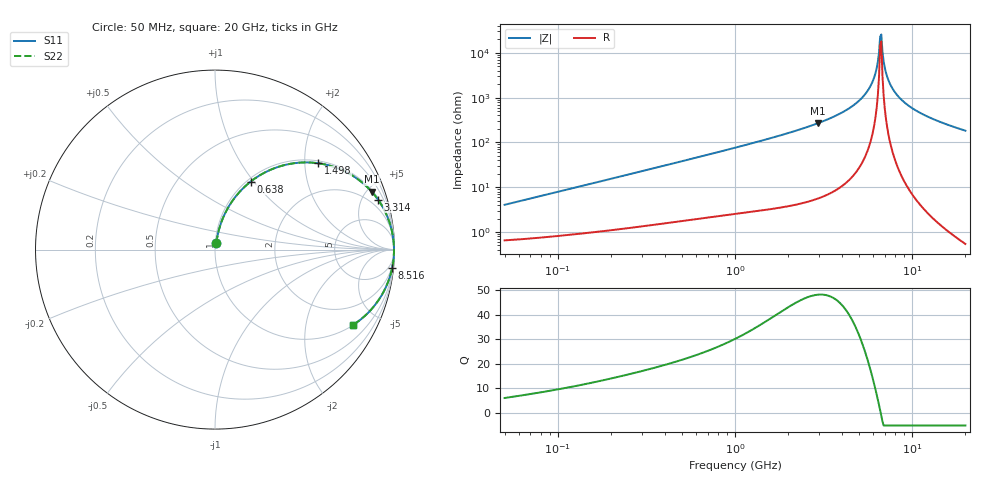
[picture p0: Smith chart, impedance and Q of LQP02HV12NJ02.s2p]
!Murata Part Number: LQP02HV12NJ02
!These Parameters are Measured in Series Mode Connection
!  o--[Z]--o
!Port1  Port2
!  o-------o
!Freq. Start=50[MHz] Stop=20[GHz], 401[Steps]
# Hz S RI R 50
!Freq.(Hz) S11(Real) S11(Imag) S21(Real) S21(Imag) S12(Real) S12(Imag) S22(Real) S22(Imag)
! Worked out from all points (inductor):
!   401 points, 50 MHz to 20 GHz, reference 50 ohm
!   read as one part in series: L = 12.6 nH near 51.52 MHz
!   highest Q = 48.1 at 2.94 GHz (marker M1), where L = 14.5 nH
!   self-resonance near 6.602 GHz
!   S11 on the Smith chart (normalised r, x): 50 MHz: 1.01, +0.08; 638 MHz: 1.04, +0.96; 1.498 GHz: 1.06, +2.33; 3.314 GHz: 1.14, +6.47; 8.516 GHz: 1, -20; 20 GHz: 1.01, -3.65
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5e7  0.00803 0.0394  0.992 -0.0394  0.992 -0.0394  0.00803 0.0394
1.364002e8  0.02 0.1031  0.98 -0.1031  0.98 -0.1031  0.02 0.1031
3.721004e8  0.0858 0.2549  0.9142 -0.2549  0.9142 -0.2549  0.0858 0.2549
6.380365e8  0.1987 0.3789  0.8013 -0.3789  0.8013 -0.3789  0.1987 0.3789
1e9  0.3704 0.4666  0.6296 -0.4666  0.6296 -0.4666  0.3704 0.4666
1.498439e9  0.5742 0.4812  0.4258 -0.4812  0.4258 -0.4812  0.5742 0.4812
2.728004e9  0.8479 0.3487  0.1521 -0.3487  0.1521 -0.3487  0.8479 0.3487
2.940159e9  0.873 0.3227  0.127 -0.3227  0.127 -0.3227  0.873 0.3227
3.314454e9  0.908 0.2787  0.092 -0.2787  0.092 -0.2787  0.908 0.2787
4.539627e9  0.971 0.1552  0.029 -0.1552  0.029 -0.1552  0.971 0.1552
5.515528e9  0.9908 0.0765  0.00922 -0.0765  0.00922 -0.0765  0.9908 0.0765
5.856089e9  0.9942 0.0521  0.00584 -0.0521  0.00584 -0.0521  0.9942 0.0521
6.125241e9  0.9959 0.0338  0.00412 -0.0338  0.00412 -0.0338  0.9959 0.0338
6.311513e9  0.9966 0.0217  0.00336 -0.0217  0.00336 -0.0217  0.9966 0.0217
6.503449e9  0.9971 0.00945  0.0029 -0.00945  0.0029 -0.00945  0.9971 0.00945
6.601595e9  0.9972 0.00335  0.00278 -0.00335  0.00278 -0.00335  0.9972 0.00335
6.802353e9  0.9972 -0.00885  0.00277 0.00885  0.00277 0.00885  0.9972 -0.00885
7.114996e9  0.9967 -0.0272  0.00333 0.0272  0.00333 0.0272  0.9967 -0.0272
7.442007e9  0.9954 -0.0455  0.00457 0.0455  0.00457 0.0455  0.9954 -0.0455
8.516016e9  0.9875 -0.1005  0.0125 0.1005  0.0125 0.1005  0.9875 -0.1005
1.183995e10  0.9399 -0.2339  0.0601 0.2339  0.0601 0.2339  0.9399 -0.2339
2e10  0.7687 -0.4202  0.2313 0.4202  0.2313 0.4202  0.7687 -0.4202
